(* Logix 5000 AddOnInstructionDefinition export AMCI_NXFE2_Configure; software revision 20.03 *)

ADD_ON_INSTRUCTION AMCI_NXFE2_Configure   (* revision 1.0 *)
VAR_INPUT
   capture_input : BOOL; {required}
   capture_input_active_state : BOOL; {required}
   external_input : BOOL; {required}
   external_input_active_state : BOOL; {required}
   home_input : BOOL; {required}
   home_input_active_state : BOOL; {required}
   _1_CW_limit_2_estop : INT; {required}
   CW_estop_actitve_state : BOOL; {required}
   _1_CCW_limit_2_estop : INT; {required}
   CCW_estop_active_state : BOOL; {required}
   Backplane_Home_Proximity_Enable : BOOL;
   Quadrature_Encoder_Enable : BOOL; {required}
   diagnostic_feedback_enable : BOOL;
   _0_CW_CCW_1_step_direction : BOOL; {required}
   _0_Limit_Switch_1_Marker_Pulse_home : BOOL;
   swap_32_bit_word_order : BOOL;
   disable_channel : BOOL;
   Starting_Speed : DINT; {required}
   homing_timeout : INT; {required}
END_VAR
VAR_IN_OUT
   NXFE2_output_data : _000A:NXFE2_0986AEB4:O:0; {required}
END_VAR
VAR
   command_data_block : INT[10];
        [0].15   // Mode Bit 1=Configuraiton Mode 0=Command Mode
END_VAR

ROUTINE Logic   (* ladder *)
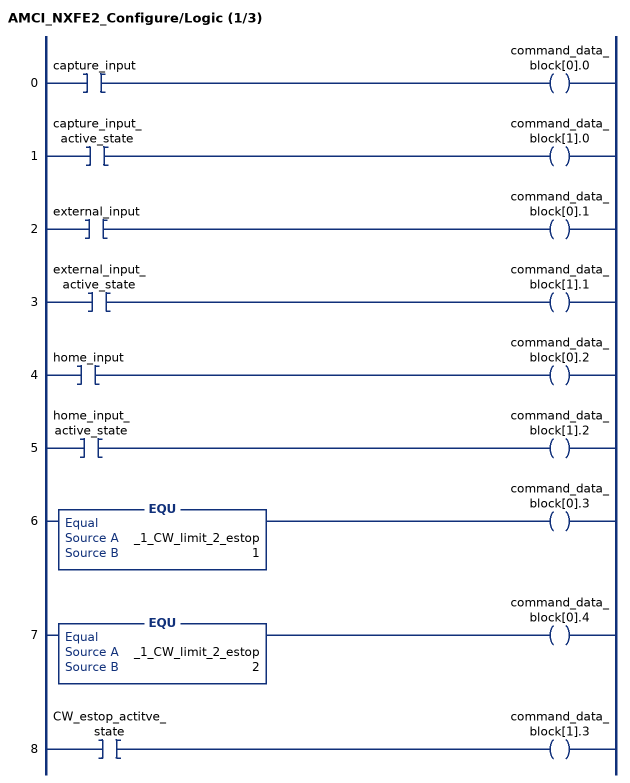
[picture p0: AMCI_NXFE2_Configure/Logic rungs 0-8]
   0: XIC(capture_input)OTE(command_data_block[0].0);
   1: XIC(capture_input_active_state)OTE(command_data_block[1].0);
   2: XIC(external_input)OTE(command_data_block[0].1);
   3: XIC(external_input_active_state)OTE(command_data_block[1].1);
   4: XIC(home_input)OTE(command_data_block[0].2);
   5: XIC(home_input_active_state)OTE(command_data_block[1].2);
   6: EQU(_1_CW_limit_2_estop,1)OTE(command_data_block[0].3);
   7: EQU(_1_CW_limit_2_estop,2)OTE(command_data_block[0].4);
   8: XIC(CW_estop_actitve_state)OTE(command_data_block[1].3);
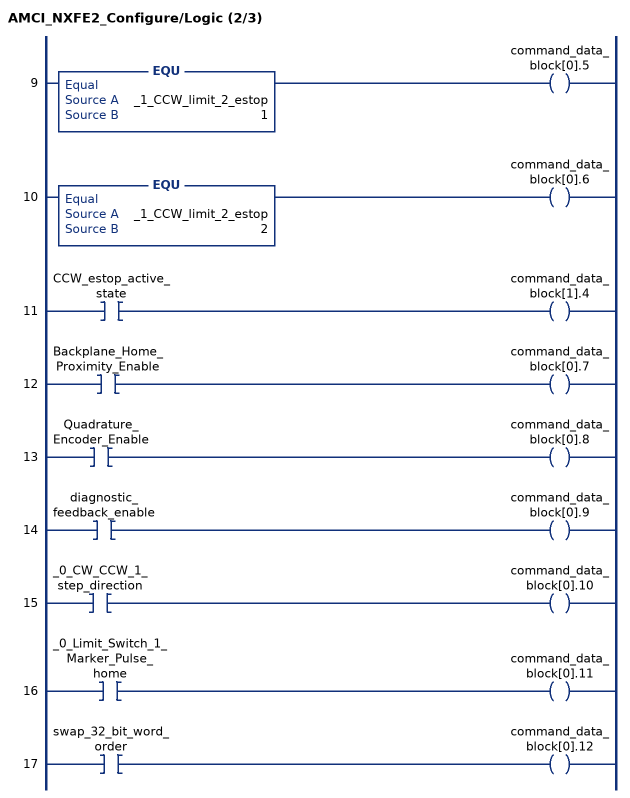
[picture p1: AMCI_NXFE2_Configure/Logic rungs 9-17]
   9: EQU(_1_CCW_limit_2_estop,1)OTE(command_data_block[0].5);
   10: EQU(_1_CCW_limit_2_estop,2)OTE(command_data_block[0].6);
   11: XIC(CCW_estop_active_state)OTE(command_data_block[1].4);
   12: XIC(Backplane_Home_Proximity_Enable)OTE(command_data_block[0].7);
   13: XIC(Quadrature_Encoder_Enable)OTE(command_data_block[0].8);
   14: XIC(diagnostic_feedback_enable)OTE(command_data_block[0].9);
   15: XIC(_0_CW_CCW_1_step_direction)OTE(command_data_block[0].10);
   16: XIC(_0_Limit_Switch_1_Marker_Pulse_home)OTE(command_data_block[0].11);
   17: XIC(swap_32_bit_word_order)OTE(command_data_block[0].12);
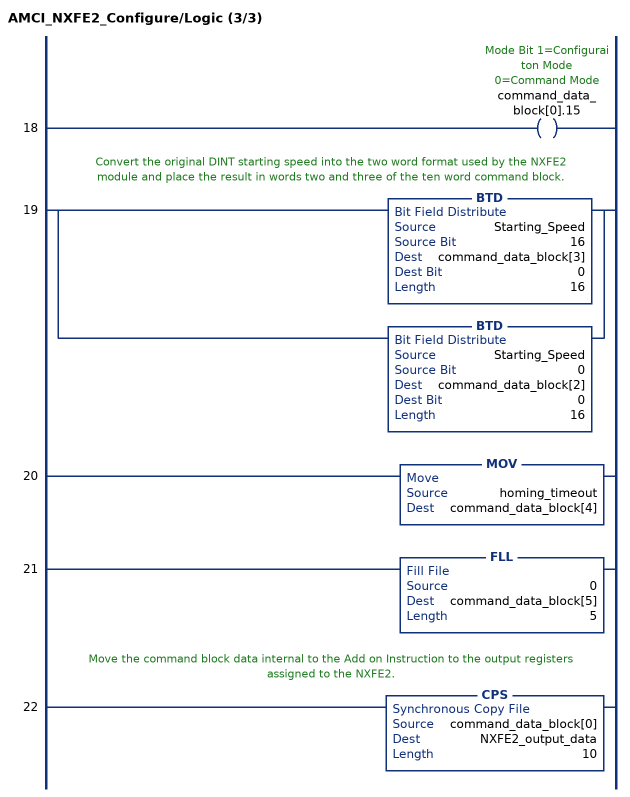
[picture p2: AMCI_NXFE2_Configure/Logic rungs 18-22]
   18: OTE(command_data_block[0].15);
   // Convert the original DINT starting speed into the two word format used by the NXFE2 module and place the result in words two and three of the ten word command block.
   19: [BTD(Starting_Speed,16,command_data_block[3],0,16) ,BTD(Starting_Speed,0,command_data_block[2],0,16) ];
   20: MOV(homing_timeout,command_data_block[4]);
   21: FLL(0,command_data_block[5],5);
   // Move the command block data internal to the Add on Instruction to the output registers assigned to the NXFE2.
   22: CPS(command_data_block[0],NXFE2_output_data,10);
END_ROUTINE
END_ADD_ON_INSTRUCTION
